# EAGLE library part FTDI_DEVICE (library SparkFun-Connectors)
Connector which mates to FTDI basic or FTDI cable.
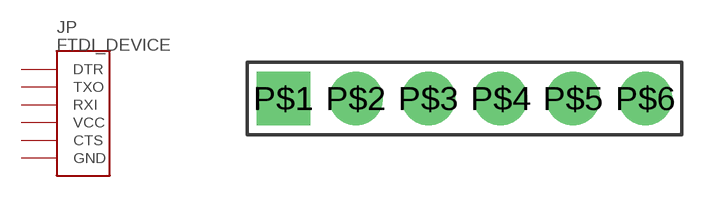
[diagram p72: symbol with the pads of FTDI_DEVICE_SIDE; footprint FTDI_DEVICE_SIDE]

Designator prefix JP

## FTDI_DEVICE  [FTDI_DEVICE_SIDE]
P$1  DTR
P$2  TXO
P$3  RXI
P$4  VCC
P$5  CTS
P$6  GND

## Footprint FTDI_DEVICE_SIDE (pad centres in mm)
Package for devices meant to mate to an FTDI connector.
drill 1.016 pad 1.88 square: P$1 -6.35,0
drill 1.016 pad 1.88: P$2 -3.81,0; P$3 -1.27,0; P$4 1.27,0; P$5 3.81,0; P$6 6.35,0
